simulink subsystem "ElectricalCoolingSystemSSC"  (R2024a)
settings: Solver=VariableStepAuto  StartTime=0.0  StopTime=10.0  RelTol=1e-3
undefined symbols (not defined in the file): BattTempInit, One, Pass, pipe, pump, radiator, T_env, tank, ThrmBatt1, ThrmBatt2, ThrmBatt3, ThrmBatt4, ThrmEM1, ThrmEM2, ThrmEM3, ThrmEM4, valve
libraries: fl_lib x109, SimscapeFluids_lib x7, nesl_utility_internal x6, autolibutils x2, nesl_utility x1, sdl_lib x1
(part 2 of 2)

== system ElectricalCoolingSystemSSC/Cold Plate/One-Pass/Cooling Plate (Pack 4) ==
  Battery to plate conduction : fl_lib/Thermal/Thermal Elements/Conductive Heat Transfer  thermal_type=foundation.enum.ConstantVariableTabulated.Constant  wall_geometry=foundation.enum.ConductionWallGeometry.Planar  area=0.5*2 m^2  thickness=1 mm  d_in=0.05 m  d_out=0.1 m  L=1 m  th_cond_min=10 W/(K*m)  th_cond=205 W/(m*K)  th_cond_TLU=[413, 401, 392, 383, 371, 357, 342] W/(K*m)  temp_TLU=[200, 273, 400, 600, 800, 1000, 1200] K  T_specify=off  T_priority=None  T=0 K  T_nominal_specify=off  T_nominal_value=1  T_nominal_unit=K  Q_specify=off  Q_priority=None  Q=0 W  Q_nominal_specify=off  Q_nominal_value=1  Q_nominal_unit=W
  "Plate mass " : fl_lib/Thermal/Thermal Elements/Thermal Mass  mass_type=foundation.enum.constant_variable.constant  mass=10*2 kg  sp_heat=910 J/kg/K  mass_min=1e-6 kg  num_ports=foundation.enum.numPorts2.one  m_specify=off  m_priority=High  m=1 kg  m_nominal_specify=off  m_nominal_value=1  m_nominal_unit=kg  T_specify=on  T_priority=High  T=BattTempInit degC  T_nominal_specify=off  T_nominal_value=1  T_nominal_unit=K  Q_specify=off  Q_priority=None  Q=0 W  Q_nominal_specify=off  Q_nominal_value=1  Q_nominal_unit=W
  H1 : PMIOPort  Side=Left
  T4 : PMIOPort  Port=2  Side=Right
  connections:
  T4/RConn1 -- Battery to plate conduction/LConn1
  "Plate mass "/LConn1 -- H1/RConn1 -- Battery to plate conduction/RConn1

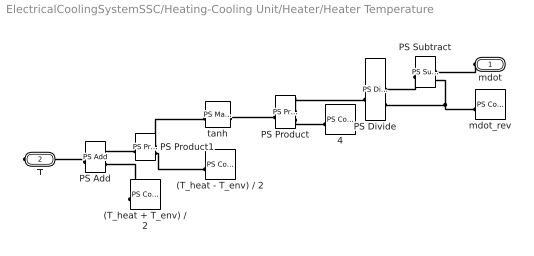
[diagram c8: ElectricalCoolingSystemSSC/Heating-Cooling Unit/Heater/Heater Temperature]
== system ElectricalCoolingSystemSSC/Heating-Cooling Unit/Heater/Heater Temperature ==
  (T_heat + T_env) / 2 : fl_lib/Physical Signals/Sources/PS Constant  constant=(T_heat +T_env + 273.15)/2 K
  (T_heat - T_env) / 2 : fl_lib/Physical Signals/Sources/PS Constant  constant=(T_heat - T_env - 273.15)/2 K
  4 : fl_lib/Physical Signals/Sources/PS Constant  constant=4
  PS Add : fl_lib/Physical Signals/Functions/PS Add
  PS Divide : fl_lib/Physical Signals/Functions/PS Divide
  PS Product : fl_lib/Physical Signals/Functions/PS Product
  PS Product1 : fl_lib/Physical Signals/Functions/PS Product
  PS Subtract : fl_lib/Physical Signals/Functions/PS Subtract
  mdot_rev : fl_lib/Physical Signals/Sources/PS Constant  constant=mdot_rev kg/s
  tanh : fl_lib/Physical Signals/Functions/PS Math Function  fcn_choice=foundation.enum.math_function.tanh  v=1
  mdot : PMIOPort  Side=Left
  T : PMIOPort  Port=2  Side=Right
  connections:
  PS Add/RConn1 -- T/RConn1
  tanh/LConn1 -- PS Product/RConn1
  PS Divide/LConn2 -- PS Subtract/LConn2 -- mdot_rev/RConn1
  PS Product/LConn2 -- 4/RConn1
  PS Add/LConn1 -- PS Product1/RConn1
  PS Subtract/RConn1 -- PS Divide/LConn1
  PS Product1/LConn2 -- (T_heat - T_env) / 2/RConn1
  PS Product1/LConn1 -- tanh/RConn1
  PS Product/LConn1 -- PS Divide/RConn1
  (T_heat + T_env) / 2/RConn1 -- PS Add/LConn2
  mdot/RConn1 -- PS Subtract/LConn1

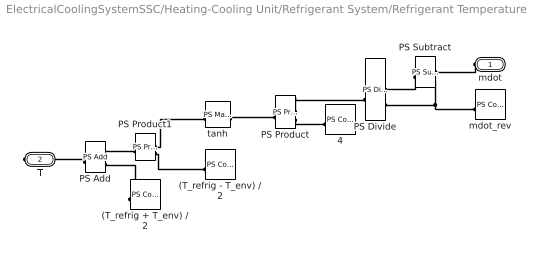
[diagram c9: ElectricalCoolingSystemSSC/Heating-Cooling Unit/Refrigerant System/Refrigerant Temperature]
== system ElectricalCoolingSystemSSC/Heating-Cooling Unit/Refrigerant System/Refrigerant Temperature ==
  (T_refrig + T_env) / 2 : fl_lib/Physical Signals/Sources/PS Constant  constant=(T_refrig+T_env+273.15)/2 K
  (T_refrig - T_env) / 2 : fl_lib/Physical Signals/Sources/PS Constant  constant=(T_refrig-T_env-273.15)/2 K
  4 : fl_lib/Physical Signals/Sources/PS Constant  constant=4
  PS Add : fl_lib/Physical Signals/Functions/PS Add
  PS Divide : fl_lib/Physical Signals/Functions/PS Divide
  PS Product : fl_lib/Physical Signals/Functions/PS Product
  PS Product1 : fl_lib/Physical Signals/Functions/PS Product
  PS Subtract : fl_lib/Physical Signals/Functions/PS Subtract
  mdot_rev : fl_lib/Physical Signals/Sources/PS Constant  constant=mdot_rev kg/s
  tanh : fl_lib/Physical Signals/Functions/PS Math Function  fcn_choice=foundation.enum.math_function.tanh  v=1
  mdot : PMIOPort  Side=Left
  T : PMIOPort  Port=2  Side=Right
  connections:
  tanh/LConn1 -- PS Product/RConn1
  PS Product/LConn1 -- PS Divide/RConn1
  (T_refrig + T_env) / 2/RConn1 -- PS Add/LConn2
  PS Divide/LConn2 -- PS Subtract/LConn2 -- mdot_rev/RConn1
  PS Add/RConn1 -- T/RConn1
  PS Add/LConn1 -- PS Product1/RConn1
  PS Product1/LConn1 -- tanh/RConn1
  PS Product/LConn2 -- 4/RConn1
  PS Subtract/RConn1 -- PS Divide/LConn1
  PS Product1/LConn2 -- (T_refrig - T_env) / 2/RConn1
  mdot/RConn1 -- PS Subtract/LConn1

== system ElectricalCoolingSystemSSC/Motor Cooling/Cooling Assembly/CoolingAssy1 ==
  Cooling Jacket1 : Subsystem
  Pipe (TL) : fl_lib/Thermal Liquid/Elements/Pipe (TL)  length=pipe.length cm  area=pipe.area cm^2  Dh=pipe.Dh cm  length_add=0 m  roughness=15e-6 m  Re_lam=2000  Re_tur=4000  shape_factor=64  Nu_lam=3.66  dynamic_compressibility=simscape.enum.onoff.off  inertia=simscape.enum.onoff.off  p0=0.101325 MPa  T0=BattTempInit degC  mdot0=0 kg/s
  H1 : PMIOPort  Side=Right
  A : PMIOPort  Port=2  Side=Left
  B : PMIOPort  Port=3  Side=Right
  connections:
  B/RConn1 -- Pipe (TL)/RConn1
  A/RConn1 -- Pipe (TL)/LConn1
  Pipe (TL)/LConn2 -- Cooling Jacket1/LConn1
  Cooling Jacket1/RConn1 -- H1/RConn1

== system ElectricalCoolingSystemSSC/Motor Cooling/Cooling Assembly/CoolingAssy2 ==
  Cooling Jacket1 : Subsystem
  Cooling Jacket2 : Subsystem
  Pipe (TL) : fl_lib/Thermal Liquid/Elements/Pipe (TL)  length=pipe.length cm  area=pipe.area cm^2  Dh=pipe.Dh cm  length_add=0 m  roughness=15e-6 m  Re_lam=2000  Re_tur=4000  shape_factor=64  Nu_lam=3.66  dynamic_compressibility=simscape.enum.onoff.off  inertia=simscape.enum.onoff.off  p0=0.101325 MPa  T0=BattTempInit degC  mdot0=0 kg/s
  Pipe (TL)1 : fl_lib/Thermal Liquid/Elements/Pipe (TL)  length=pipe.length cm  area=pipe.area cm^2  Dh=pipe.Dh cm  length_add=0 m  roughness=15e-6 m  Re_lam=2000  Re_tur=4000  shape_factor=64  Nu_lam=3.66  dynamic_compressibility=simscape.enum.onoff.off  inertia=simscape.enum.onoff.off  p0=0.101325 MPa  T0=BattTempInit degC  mdot0=0 kg/s
  A : PMIOPort  Side=Left
  H2 : PMIOPort  Port=2  Side=Right
  H1 : PMIOPort  Port=3  Side=Right
  B : PMIOPort  Port=4  Side=Right
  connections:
  Pipe (TL)1/LConn2 -- Cooling Jacket2/LConn1
  Cooling Jacket2/RConn1 -- H2/RConn1
  B/RConn1 -- Pipe (TL)1/RConn1
  A/RConn1 -- Pipe (TL)/LConn1
  Cooling Jacket1/LConn1 -- Pipe (TL)/LConn2
  H1/RConn1 -- Cooling Jacket1/RConn1
  Pipe (TL)/RConn1 -- Pipe (TL)1/LConn1

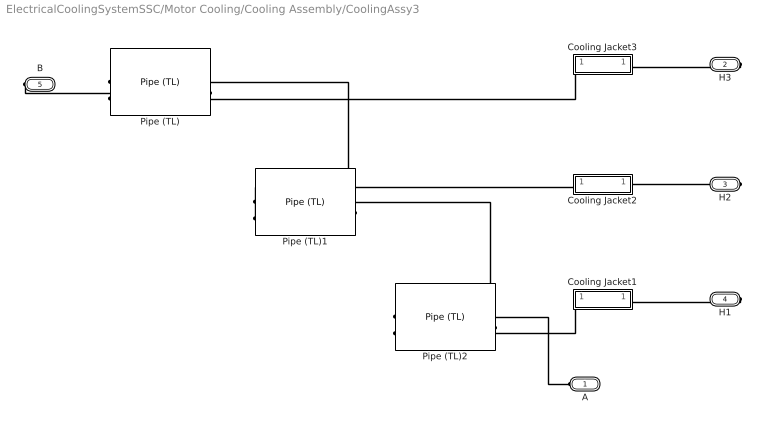
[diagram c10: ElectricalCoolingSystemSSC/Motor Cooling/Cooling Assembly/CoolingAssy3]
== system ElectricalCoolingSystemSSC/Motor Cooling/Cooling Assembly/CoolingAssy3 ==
  Cooling Jacket1 : Subsystem
  Cooling Jacket2 : Subsystem
  Cooling Jacket3 : Subsystem
  Pipe (TL) : fl_lib/Thermal Liquid/Elements/Pipe (TL)  length=pipe.length cm  area=pipe.area cm^2  Dh=pipe.Dh cm  length_add=0 m  roughness=15e-6 m  Re_lam=2000  Re_tur=4000  shape_factor=64  Nu_lam=3.66  dynamic_compressibility=simscape.enum.onoff.off  inertia=simscape.enum.onoff.off  p0=0.101325 MPa  T0=BattTempInit degC  mdot0=0 kg/s
  Pipe (TL)1 : fl_lib/Thermal Liquid/Elements/Pipe (TL)  length=pipe.length cm  area=pipe.area cm^2  Dh=pipe.Dh cm  length_add=0 m  roughness=15e-6 m  Re_lam=2000  Re_tur=4000  shape_factor=64  Nu_lam=3.66  dynamic_compressibility=simscape.enum.onoff.off  inertia=simscape.enum.onoff.off  p0=0.101325 MPa  T0=BattTempInit degC  mdot0=0 kg/s
  Pipe (TL)2 : fl_lib/Thermal Liquid/Elements/Pipe (TL)  length=pipe.length cm  area=pipe.area cm^2  Dh=pipe.Dh cm  length_add=0 m  roughness=15e-6 m  Re_lam=2000  Re_tur=4000  shape_factor=64  Nu_lam=3.66  dynamic_compressibility=simscape.enum.onoff.off  inertia=simscape.enum.onoff.off  p0=0.101325 MPa  T0=BattTempInit degC  mdot0=0 kg/s
  A : PMIOPort  Side=Left
  H3 : PMIOPort  Port=2  Side=Right
  H2 : PMIOPort  Port=3  Side=Right
  H1 : PMIOPort  Port=4  Side=Right
  B : PMIOPort  Port=5  Side=Right
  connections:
  Cooling Jacket3/LConn1 -- Pipe (TL)/LConn2
  B/RConn1 -- Pipe (TL)/RConn1
  H3/RConn1 -- Cooling Jacket3/RConn1
  Pipe (TL)1/LConn2 -- Cooling Jacket2/LConn1
  Cooling Jacket2/RConn1 -- H2/RConn1
  A/RConn1 -- Pipe (TL)2/LConn1
  Cooling Jacket1/LConn1 -- Pipe (TL)2/LConn2
  H1/RConn1 -- Cooling Jacket1/RConn1
  Pipe (TL)2/RConn1 -- Pipe (TL)1/LConn1
  Pipe (TL)1/RConn1 -- Pipe (TL)/LConn1

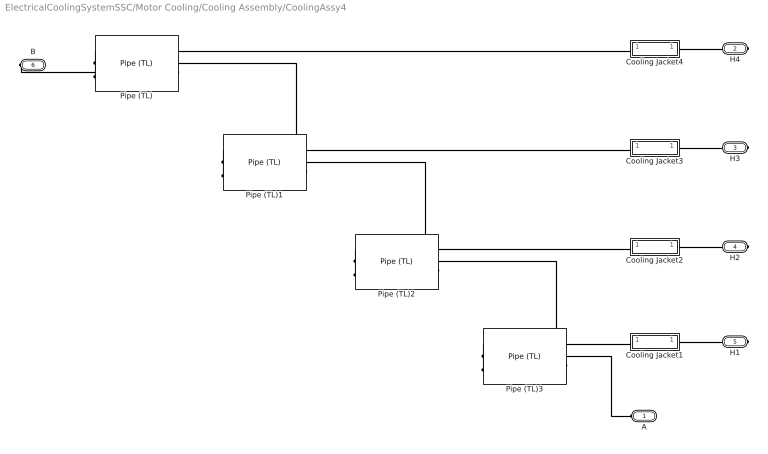
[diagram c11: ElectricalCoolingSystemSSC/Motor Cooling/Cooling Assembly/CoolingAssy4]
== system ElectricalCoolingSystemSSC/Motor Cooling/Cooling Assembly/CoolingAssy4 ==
  Cooling Jacket1 : Subsystem
  Cooling Jacket2 : Subsystem
  Cooling Jacket3 : Subsystem
  Cooling Jacket4 : Subsystem
  Pipe (TL){,1..3} (4 alike) : fl_lib/Thermal Liquid/Elements/Pipe (TL)  length=pipe.length cm  area=pipe.area cm^2  Dh=pipe.Dh cm  length_add=0 m  roughness=15e-6 m  Re_lam=2000  Re_tur=4000  shape_factor=64  Nu_lam=3.66  dynamic_compressibility=simscape.enum.onoff.off  inertia=simscape.enum.onoff.off  p0=0.101325 MPa  T0=BattTempInit degC  mdot0=0 kg/s
  A : PMIOPort  Side=Left
  H4 : PMIOPort  Port=2  Side=Right
  H3 : PMIOPort  Port=3  Side=Right
  H2 : PMIOPort  Port=4  Side=Right
  H1 : PMIOPort  Port=5  Side=Right
  B : PMIOPort  Port=6  Side=Right
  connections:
  Pipe (TL)/LConn2 -- Cooling Jacket4/LConn1
  Cooling Jacket4/RConn1 -- H4/RConn1
  B/RConn1 -- Pipe (TL)/RConn1
  Pipe (TL)1/LConn2 -- Cooling Jacket3/LConn1
  Cooling Jacket3/RConn1 -- H3/RConn1
  Pipe (TL)2/LConn2 -- Cooling Jacket2/LConn1
  Cooling Jacket2/RConn1 -- H2/RConn1
  A/RConn1 -- Pipe (TL)3/LConn1
  Pipe (TL)3/LConn2 -- Cooling Jacket1/LConn1
  Cooling Jacket1/RConn1 -- H1/RConn1
  Pipe (TL)3/RConn1 -- Pipe (TL)2/LConn1
  Pipe (TL)2/RConn1 -- Pipe (TL)1/LConn1
  Pipe (TL)1/RConn1 -- Pipe (TL)/LConn1

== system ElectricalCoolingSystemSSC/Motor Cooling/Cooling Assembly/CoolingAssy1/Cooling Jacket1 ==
  Conduction : fl_lib/Thermal/Thermal Elements/Conductive Heat Transfer  thermal_type=foundation.enum.ConstantVariableTabulated.Constant  wall_geometry=foundation.enum.ConductionWallGeometry.Planar  area=0.5*2 m^2  thickness=1 mm  d_in=0.05 m  d_out=0.1 m  L=1 m  th_cond_min=10 W/(K*m)  th_cond=205 W/(m*K)  th_cond_TLU=[413, 401, 392, 383, 371, 357, 342] W/(K*m)  temp_TLU=[200, 273, 400, 600, 800, 1000, 1200] K  T_specify=off  T_priority=None  T=0 K  T_nominal_specify=off  T_nominal_value=1  T_nominal_unit=K  Q_specify=off  Q_priority=None  Q=0 W  Q_nominal_specify=off  Q_nominal_value=1  Q_nominal_unit=W
  "Mass " : fl_lib/Thermal/Thermal Elements/Thermal Mass  mass_type=foundation.enum.constant_variable.constant  mass=10 kg  sp_heat=890 J/kg/K  mass_min=1e-6 kg  num_ports=foundation.enum.numPorts2.one  m_specify=off  m_priority=High  m=1 kg  m_nominal_specify=off  m_nominal_value=1  m_nominal_unit=kg  T_specify=on  T_priority=High  T=BattTempInit degC  T_nominal_specify=off  T_nominal_value=1  T_nominal_unit=K  Q_specify=off  Q_priority=None  Q=0 W  Q_nominal_specify=off  Q_nominal_value=1  Q_nominal_unit=W
  H1 : PMIOPort  Side=Left
  T1 : PMIOPort  Port=2  Side=Right
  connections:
  Conduction/LConn1 -- T1/RConn1
  Conduction/RConn1 -- H1/RConn1 -- "Mass "/LConn1

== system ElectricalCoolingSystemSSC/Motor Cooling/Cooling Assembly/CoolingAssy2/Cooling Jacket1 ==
  Conduction : fl_lib/Thermal/Thermal Elements/Conductive Heat Transfer  thermal_type=foundation.enum.ConstantVariableTabulated.Constant  wall_geometry=foundation.enum.ConductionWallGeometry.Planar  area=0.5*2 m^2  thickness=1 mm  d_in=0.05 m  d_out=0.1 m  L=1 m  th_cond_min=10 W/(K*m)  th_cond=205 W/(m*K)  th_cond_TLU=[413, 401, 392, 383, 371, 357, 342] W/(K*m)  temp_TLU=[200, 273, 400, 600, 800, 1000, 1200] K  T_specify=off  T_priority=None  T=0 K  T_nominal_specify=off  T_nominal_value=1  T_nominal_unit=K  Q_specify=off  Q_priority=None  Q=0 W  Q_nominal_specify=off  Q_nominal_value=1  Q_nominal_unit=W
  "Mass " : fl_lib/Thermal/Thermal Elements/Thermal Mass  mass_type=foundation.enum.constant_variable.constant  mass=10 kg  sp_heat=890 J/kg/K  mass_min=1e-6 kg  num_ports=foundation.enum.numPorts2.one  m_specify=off  m_priority=High  m=1 kg  m_nominal_specify=off  m_nominal_value=1  m_nominal_unit=kg  T_specify=on  T_priority=High  T=BattTempInit degC  T_nominal_specify=off  T_nominal_value=1  T_nominal_unit=K  Q_specify=off  Q_priority=None  Q=0 W  Q_nominal_specify=off  Q_nominal_value=1  Q_nominal_unit=W
  H1 : PMIOPort  Side=Left
  T1 : PMIOPort  Port=2  Side=Right
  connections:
  Conduction/LConn1 -- T1/RConn1
  Conduction/RConn1 -- H1/RConn1 -- "Mass "/LConn1

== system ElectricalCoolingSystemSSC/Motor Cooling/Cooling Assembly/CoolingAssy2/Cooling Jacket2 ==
  Conduction : fl_lib/Thermal/Thermal Elements/Conductive Heat Transfer  thermal_type=foundation.enum.ConstantVariableTabulated.Constant  wall_geometry=foundation.enum.ConductionWallGeometry.Planar  area=0.5*2 m^2  thickness=1 mm  d_in=0.05 m  d_out=0.1 m  L=1 m  th_cond_min=10 W/(K*m)  th_cond=205 W/(m*K)  th_cond_TLU=[413, 401, 392, 383, 371, 357, 342] W/(K*m)  temp_TLU=[200, 273, 400, 600, 800, 1000, 1200] K  T_specify=off  T_priority=None  T=0 K  T_nominal_specify=off  T_nominal_value=1  T_nominal_unit=K  Q_specify=off  Q_priority=None  Q=0 W  Q_nominal_specify=off  Q_nominal_value=1  Q_nominal_unit=W
  "Mass " : fl_lib/Thermal/Thermal Elements/Thermal Mass  mass_type=foundation.enum.constant_variable.constant  mass=10 kg  sp_heat=890 J/kg/K  mass_min=1e-6 kg  num_ports=foundation.enum.numPorts2.one  m_specify=off  m_priority=High  m=1 kg  m_nominal_specify=off  m_nominal_value=1  m_nominal_unit=kg  T_specify=on  T_priority=High  T=BattTempInit degC  T_nominal_specify=off  T_nominal_value=1  T_nominal_unit=K  Q_specify=off  Q_priority=None  Q=0 W  Q_nominal_specify=off  Q_nominal_value=1  Q_nominal_unit=W
  H1 : PMIOPort  Side=Left
  T1 : PMIOPort  Port=2  Side=Right
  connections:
  Conduction/LConn1 -- T1/RConn1
  Conduction/RConn1 -- H1/RConn1 -- "Mass "/LConn1

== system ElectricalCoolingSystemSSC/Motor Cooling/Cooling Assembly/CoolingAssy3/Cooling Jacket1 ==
  Conduction : fl_lib/Thermal/Thermal Elements/Conductive Heat Transfer  thermal_type=foundation.enum.ConstantVariableTabulated.Constant  wall_geometry=foundation.enum.ConductionWallGeometry.Planar  area=0.5*2 m^2  thickness=1 mm  d_in=0.05 m  d_out=0.1 m  L=1 m  th_cond_min=10 W/(K*m)  th_cond=205 W/(m*K)  th_cond_TLU=[413, 401, 392, 383, 371, 357, 342] W/(K*m)  temp_TLU=[200, 273, 400, 600, 800, 1000, 1200] K  T_specify=off  T_priority=None  T=0 K  T_nominal_specify=off  T_nominal_value=1  T_nominal_unit=K  Q_specify=off  Q_priority=None  Q=0 W  Q_nominal_specify=off  Q_nominal_value=1  Q_nominal_unit=W
  "Mass " : fl_lib/Thermal/Thermal Elements/Thermal Mass  mass_type=foundation.enum.constant_variable.constant  mass=10 kg  sp_heat=890 J/kg/K  mass_min=1e-6 kg  num_ports=foundation.enum.numPorts2.one  m_specify=off  m_priority=High  m=1 kg  m_nominal_specify=off  m_nominal_value=1  m_nominal_unit=kg  T_specify=on  T_priority=High  T=BattTempInit degC  T_nominal_specify=off  T_nominal_value=1  T_nominal_unit=K  Q_specify=off  Q_priority=None  Q=0 W  Q_nominal_specify=off  Q_nominal_value=1  Q_nominal_unit=W
  H1 : PMIOPort  Side=Left
  T1 : PMIOPort  Port=2  Side=Right
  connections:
  Conduction/LConn1 -- T1/RConn1
  Conduction/RConn1 -- H1/RConn1 -- "Mass "/LConn1

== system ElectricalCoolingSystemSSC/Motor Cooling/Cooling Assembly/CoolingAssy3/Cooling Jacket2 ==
  Conduction : fl_lib/Thermal/Thermal Elements/Conductive Heat Transfer  thermal_type=foundation.enum.ConstantVariableTabulated.Constant  wall_geometry=foundation.enum.ConductionWallGeometry.Planar  area=0.5*2 m^2  thickness=1 mm  d_in=0.05 m  d_out=0.1 m  L=1 m  th_cond_min=10 W/(K*m)  th_cond=205 W/(m*K)  th_cond_TLU=[413, 401, 392, 383, 371, 357, 342] W/(K*m)  temp_TLU=[200, 273, 400, 600, 800, 1000, 1200] K  T_specify=off  T_priority=None  T=0 K  T_nominal_specify=off  T_nominal_value=1  T_nominal_unit=K  Q_specify=off  Q_priority=None  Q=0 W  Q_nominal_specify=off  Q_nominal_value=1  Q_nominal_unit=W
  "Mass " : fl_lib/Thermal/Thermal Elements/Thermal Mass  mass_type=foundation.enum.constant_variable.constant  mass=10 kg  sp_heat=890 J/kg/K  mass_min=1e-6 kg  num_ports=foundation.enum.numPorts2.one  m_specify=off  m_priority=High  m=1 kg  m_nominal_specify=off  m_nominal_value=1  m_nominal_unit=kg  T_specify=on  T_priority=High  T=BattTempInit degC  T_nominal_specify=off  T_nominal_value=1  T_nominal_unit=K  Q_specify=off  Q_priority=None  Q=0 W  Q_nominal_specify=off  Q_nominal_value=1  Q_nominal_unit=W
  H1 : PMIOPort  Side=Left
  T1 : PMIOPort  Port=2  Side=Right
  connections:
  Conduction/LConn1 -- T1/RConn1
  Conduction/RConn1 -- H1/RConn1 -- "Mass "/LConn1

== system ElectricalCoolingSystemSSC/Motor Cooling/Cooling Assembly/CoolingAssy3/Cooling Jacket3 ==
  Conduction : fl_lib/Thermal/Thermal Elements/Conductive Heat Transfer  thermal_type=foundation.enum.ConstantVariableTabulated.Constant  wall_geometry=foundation.enum.ConductionWallGeometry.Planar  area=0.5*2 m^2  thickness=1 mm  d_in=0.05 m  d_out=0.1 m  L=1 m  th_cond_min=10 W/(K*m)  th_cond=205 W/(m*K)  th_cond_TLU=[413, 401, 392, 383, 371, 357, 342] W/(K*m)  temp_TLU=[200, 273, 400, 600, 800, 1000, 1200] K  T_specify=off  T_priority=None  T=0 K  T_nominal_specify=off  T_nominal_value=1  T_nominal_unit=K  Q_specify=off  Q_priority=None  Q=0 W  Q_nominal_specify=off  Q_nominal_value=1  Q_nominal_unit=W
  "Mass " : fl_lib/Thermal/Thermal Elements/Thermal Mass  mass_type=foundation.enum.constant_variable.constant  mass=10 kg  sp_heat=890 J/kg/K  mass_min=1e-6 kg  num_ports=foundation.enum.numPorts2.one  m_specify=off  m_priority=High  m=1 kg  m_nominal_specify=off  m_nominal_value=1  m_nominal_unit=kg  T_specify=on  T_priority=High  T=BattTempInit degC  T_nominal_specify=off  T_nominal_value=1  T_nominal_unit=K  Q_specify=off  Q_priority=None  Q=0 W  Q_nominal_specify=off  Q_nominal_value=1  Q_nominal_unit=W
  H1 : PMIOPort  Side=Left
  T1 : PMIOPort  Port=2  Side=Right
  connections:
  Conduction/LConn1 -- T1/RConn1
  Conduction/RConn1 -- H1/RConn1 -- "Mass "/LConn1

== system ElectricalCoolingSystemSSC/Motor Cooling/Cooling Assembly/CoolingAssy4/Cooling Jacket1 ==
  Conduction : fl_lib/Thermal/Thermal Elements/Conductive Heat Transfer  thermal_type=foundation.enum.ConstantVariableTabulated.Constant  wall_geometry=foundation.enum.ConductionWallGeometry.Planar  area=0.5*2 m^2  thickness=1 mm  d_in=0.05 m  d_out=0.1 m  L=1 m  th_cond_min=10 W/(K*m)  th_cond=205 W/(m*K)  th_cond_TLU=[413, 401, 392, 383, 371, 357, 342] W/(K*m)  temp_TLU=[200, 273, 400, 600, 800, 1000, 1200] K  T_specify=off  T_priority=None  T=0 K  T_nominal_specify=off  T_nominal_value=1  T_nominal_unit=K  Q_specify=off  Q_priority=None  Q=0 W  Q_nominal_specify=off  Q_nominal_value=1  Q_nominal_unit=W
  "Mass " : fl_lib/Thermal/Thermal Elements/Thermal Mass  mass_type=foundation.enum.constant_variable.constant  mass=10 kg  sp_heat=890 J/kg/K  mass_min=1e-6 kg  num_ports=foundation.enum.numPorts2.one  m_specify=off  m_priority=High  m=1 kg  m_nominal_specify=off  m_nominal_value=1  m_nominal_unit=kg  T_specify=on  T_priority=High  T=BattTempInit degC  T_nominal_specify=off  T_nominal_value=1  T_nominal_unit=K  Q_specify=off  Q_priority=None  Q=0 W  Q_nominal_specify=off  Q_nominal_value=1  Q_nominal_unit=W
  H1 : PMIOPort  Side=Left
  T1 : PMIOPort  Port=2  Side=Right
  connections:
  Conduction/LConn1 -- T1/RConn1
  Conduction/RConn1 -- H1/RConn1 -- "Mass "/LConn1

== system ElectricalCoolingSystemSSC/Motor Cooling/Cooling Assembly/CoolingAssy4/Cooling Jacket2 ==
  Conduction : fl_lib/Thermal/Thermal Elements/Conductive Heat Transfer  thermal_type=foundation.enum.ConstantVariableTabulated.Constant  wall_geometry=foundation.enum.ConductionWallGeometry.Planar  area=0.5*2 m^2  thickness=1 mm  d_in=0.05 m  d_out=0.1 m  L=1 m  th_cond_min=10 W/(K*m)  th_cond=205 W/(m*K)  th_cond_TLU=[413, 401, 392, 383, 371, 357, 342] W/(K*m)  temp_TLU=[200, 273, 400, 600, 800, 1000, 1200] K  T_specify=off  T_priority=None  T=0 K  T_nominal_specify=off  T_nominal_value=1  T_nominal_unit=K  Q_specify=off  Q_priority=None  Q=0 W  Q_nominal_specify=off  Q_nominal_value=1  Q_nominal_unit=W
  "Mass " : fl_lib/Thermal/Thermal Elements/Thermal Mass  mass_type=foundation.enum.constant_variable.constant  mass=10 kg  sp_heat=890 J/kg/K  mass_min=1e-6 kg  num_ports=foundation.enum.numPorts2.one  m_specify=off  m_priority=High  m=1 kg  m_nominal_specify=off  m_nominal_value=1  m_nominal_unit=kg  T_specify=on  T_priority=High  T=BattTempInit degC  T_nominal_specify=off  T_nominal_value=1  T_nominal_unit=K  Q_specify=off  Q_priority=None  Q=0 W  Q_nominal_specify=off  Q_nominal_value=1  Q_nominal_unit=W
  H1 : PMIOPort  Side=Left
  T1 : PMIOPort  Port=2  Side=Right
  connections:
  Conduction/LConn1 -- T1/RConn1
  Conduction/RConn1 -- H1/RConn1 -- "Mass "/LConn1

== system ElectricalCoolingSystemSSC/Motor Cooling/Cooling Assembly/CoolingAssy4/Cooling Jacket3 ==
  Conduction : fl_lib/Thermal/Thermal Elements/Conductive Heat Transfer  thermal_type=foundation.enum.ConstantVariableTabulated.Constant  wall_geometry=foundation.enum.ConductionWallGeometry.Planar  area=0.5*2 m^2  thickness=1 mm  d_in=0.05 m  d_out=0.1 m  L=1 m  th_cond_min=10 W/(K*m)  th_cond=205 W/(m*K)  th_cond_TLU=[413, 401, 392, 383, 371, 357, 342] W/(K*m)  temp_TLU=[200, 273, 400, 600, 800, 1000, 1200] K  T_specify=off  T_priority=None  T=0 K  T_nominal_specify=off  T_nominal_value=1  T_nominal_unit=K  Q_specify=off  Q_priority=None  Q=0 W  Q_nominal_specify=off  Q_nominal_value=1  Q_nominal_unit=W
  "Mass " : fl_lib/Thermal/Thermal Elements/Thermal Mass  mass_type=foundation.enum.constant_variable.constant  mass=10 kg  sp_heat=890 J/kg/K  mass_min=1e-6 kg  num_ports=foundation.enum.numPorts2.one  m_specify=off  m_priority=High  m=1 kg  m_nominal_specify=off  m_nominal_value=1  m_nominal_unit=kg  T_specify=on  T_priority=High  T=BattTempInit degC  T_nominal_specify=off  T_nominal_value=1  T_nominal_unit=K  Q_specify=off  Q_priority=None  Q=0 W  Q_nominal_specify=off  Q_nominal_value=1  Q_nominal_unit=W
  H1 : PMIOPort  Side=Left
  T1 : PMIOPort  Port=2  Side=Right
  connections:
  Conduction/LConn1 -- T1/RConn1
  Conduction/RConn1 -- H1/RConn1 -- "Mass "/LConn1

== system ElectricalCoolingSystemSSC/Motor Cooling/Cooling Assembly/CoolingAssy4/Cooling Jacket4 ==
  Conduction : fl_lib/Thermal/Thermal Elements/Conductive Heat Transfer  thermal_type=foundation.enum.ConstantVariableTabulated.Constant  wall_geometry=foundation.enum.ConductionWallGeometry.Planar  area=0.5*2 m^2  thickness=1 mm  d_in=0.05 m  d_out=0.1 m  L=1 m  th_cond_min=10 W/(K*m)  th_cond=205 W/(m*K)  th_cond_TLU=[413, 401, 392, 383, 371, 357, 342] W/(K*m)  temp_TLU=[200, 273, 400, 600, 800, 1000, 1200] K  T_specify=off  T_priority=None  T=0 K  T_nominal_specify=off  T_nominal_value=1  T_nominal_unit=K  Q_specify=off  Q_priority=None  Q=0 W  Q_nominal_specify=off  Q_nominal_value=1  Q_nominal_unit=W
  "Mass " : fl_lib/Thermal/Thermal Elements/Thermal Mass  mass_type=foundation.enum.constant_variable.constant  mass=10 kg  sp_heat=890 J/kg/K  mass_min=1e-6 kg  num_ports=foundation.enum.numPorts2.one  m_specify=off  m_priority=High  m=1 kg  m_nominal_specify=off  m_nominal_value=1  m_nominal_unit=kg  T_specify=on  T_priority=High  T=BattTempInit degC  T_nominal_specify=off  T_nominal_value=1  T_nominal_unit=K  Q_specify=off  Q_priority=None  Q=0 W  Q_nominal_specify=off  Q_nominal_value=1  Q_nominal_unit=W
  H1 : PMIOPort  Side=Left
  T1 : PMIOPort  Port=2  Side=Right
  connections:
  Conduction/LConn1 -- T1/RConn1
  Conduction/RConn1 -- H1/RConn1 -- "Mass "/LConn1
